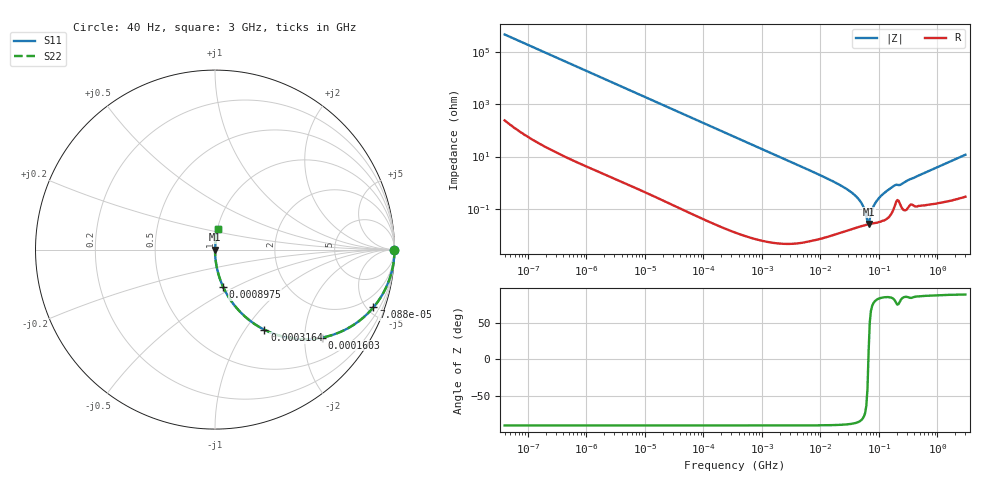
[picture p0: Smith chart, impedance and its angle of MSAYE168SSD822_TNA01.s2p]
! MSAYE168SSD822_TNA01  S-PARAMETER MODEL  ( General Type )
! Model Generated by TAIYO YUDEN Corporation (http://www.ty-top.com)
! Version 2.0
! TAIYO YUDEN Control No. 031107
! Copyright(c) 2003 TAIYO YUDEN CO.,LTD. All Rights Reserved.
! Product Description (link to TY-COMPAS)
! https://ds.yuden.co.jp/TYCOMPAS/or/detail?pn=MSAYE168SSD822KTNA01&u=M
! Products Name : Multilayer Ceramic Capacitors
! Characteristics :
!  Capacitance : 8200 pF , Rated Voltage : 16V
!  Case Size : 1.6 x 0.8 / 0.063 x 0.031 [mm/inch] , Thickness : 0.8 / 0.031 [mm/inch]
!  (Conditions: Temperature = 25 degC , DC Bias Current/Voltage = 0A / 0V)
! External Node Assignments :
!  1  o---| |---o  2
! GND o---------o GND
! Frequency Range : 40Hz  -  3GHz  [ 401 STEP ]
# MHz S RI R 50
! Freq[MHz].  S11 Real  S11 Imag  S21 Real  S21 Imag  S12 Real  S12 Imag  S22 Real  S22 Imag
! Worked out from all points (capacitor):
!   401 points, 40 Hz to 3 GHz, reference 50 ohm
!   read as one part in series: C = 8.17 nF near 44 Hz
!   lowest |Z| = 25.5 mohm at 66.58 MHz (marker M1)
!   series resonance near 66 MHz, so ESL is about 710 pH
!   S11 on the Smith chart (normalised r, x): 40 Hz: open; 70.88 kHz: 1.00, -5.50; 160.3 kHz: 1.00, -2.43; 316.4 kHz: 1.00, -1.23; 897.5 kHz: 1.00, -0.43; 3 GHz: 1.01, +0.23
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4e-05  1 -0.000205  1.45e-07 0.000205  1.45e-07 0.000205  1 -0.000205
0.000834  1 -0.00428  1.92e-05 0.00428  1.92e-05 0.00428  1 -0.00428
0.017386  0.9921 -0.0886  0.00792 0.0886  0.00792 0.0886  0.9921 -0.0886
0.07088  0.883 -0.3213  0.117 0.3213  0.117 0.3213  0.883 -0.3213
0.160288  0.5962 -0.4906  0.4038 0.4906  0.4038 0.4906  0.5962 -0.4906
0.316385  0.2749 -0.4463  0.7251 0.4463  0.7251 0.4463  0.2749 -0.4463
0.362475  0.2241 -0.4169  0.7759 0.4169  0.7759 0.4169  0.2241 -0.4169
0.897494  0.045 -0.2072  0.955 0.2072  0.955 0.2072  0.045 -0.2072
2.222206  0.00765 -0.0869  0.9923 0.0869  0.9923 0.0869  0.00765 -0.0869
7.222098  0.000768 -0.0266  0.9992 0.0266  0.9992 0.0266  0.000768 -0.0266
20.48705  0.000185 -0.00856  0.9998 0.00856  0.9998 0.00856  0.000185 -0.00856
36.93337  0.000185 -0.0036  0.9998 0.0036  0.9998 0.0036  0.000185 -0.0036
48.47801  0.000211 -0.00183  0.9998 0.00183  0.9998 0.00183  0.000211 -0.00183
55.54024  0.000227 -0.00101  0.9998 0.00101  0.9998 0.00101  0.000227 -0.00101
60.81113  0.000238 -0.00047  0.9998 0.00047  0.9998 0.00047  0.000238 -0.00047
66.58224  0.00025 5.07e-05  0.9997 -5.07e-05  0.9997 -5.07e-05  0.00025 5.07e-05
69.67004  0.000256 0.000314  0.9997 -0.000314  0.9997 -0.000314  0.000256 0.000314
79.8195  0.000275 0.00113  0.9997 -0.00113  0.9997 -0.00113  0.000275 0.00113
91.44753  0.000293 0.00195  0.9997 -0.00195  0.9997 -0.00195  0.000293 0.00195
150.5692  0.000527 0.00561  0.9995 -0.00561  0.9995 -0.00561  0.000527 0.00561
180.504  0.00109 0.0074  0.9989 -0.0074  0.9989 -0.0074  0.00109 0.0074
3000  0.0163 0.1149  0.9837 -0.1149  0.9837 -0.1149  0.0163 0.1149
